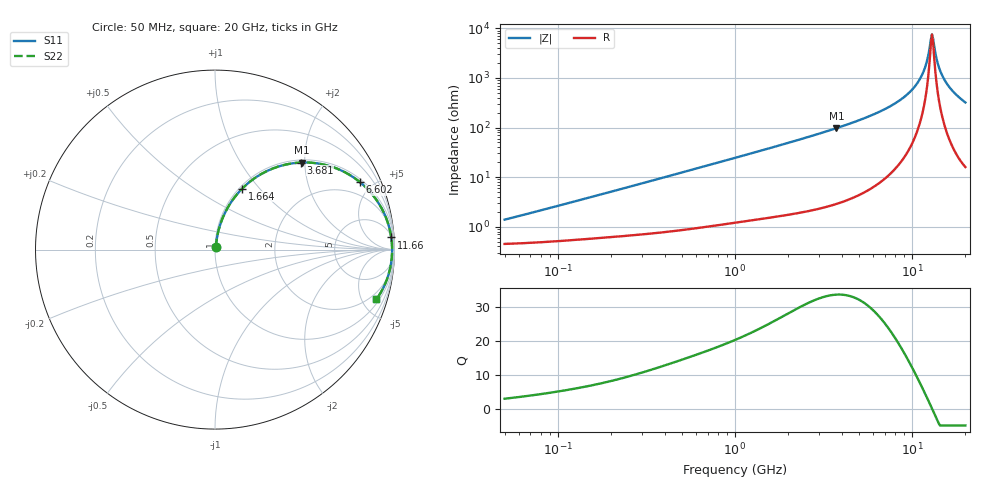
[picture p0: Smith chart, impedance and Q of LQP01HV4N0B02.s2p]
!Murata Part Number: LQP01HV4N0B02
!These Parameters are Measured in Series Mode Connection
!  o--[Z]--o
!Port1  Port2
!  o-------o
!Freq. Start=50[MHz] Stop=20[GHz], 401[Steps]
# Hz S RI R 50
!Freq.(Hz) S11(Real) S11(Imag) S21(Real) S21(Imag) S12(Real) S12(Imag) S22(Real) S22(Imag)
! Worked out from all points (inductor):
!   401 points, 50 MHz to 20 GHz, reference 50 ohm
!   read as one part in series: L = 4.16 nH near 52.3 MHz
!   highest Q = 33.8 at 3.736 GHz (marker M1), where L = 4.13 nH
!   self-resonance near 12.95 GHz
!   S11 on the Smith chart (normalised r, x): 50 MHz: 1.01, +0.03; 1.664 GHz: 1.03, +0.81; 3.681 GHz: 1.06, +1.91; 6.602 GHz: 1.16, +4.22; 11.66 GHz: 6, +28; 20 GHz: 1.32, -6.39
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5e7  0.00465 0.013  0.9954 -0.013  0.9954 -0.013  0.00465 0.013
1.364002e8  0.00671 0.0345  0.9933 -0.0345  0.9933 -0.0345  0.00671 0.0345
3.721004e8  0.0158 0.0903  0.9842 -0.0903  0.9842 -0.0903  0.0158 0.0903
1e9  0.0663 0.2253  0.9337 -0.2253  0.9337 -0.2253  0.0663 0.2253
1.664083e9  0.1515 0.3398  0.8485 -0.3398  0.8485 -0.3398  0.1515 0.3398
2.728004e9  0.3227 0.4521  0.6773 -0.4521  0.6773 -0.4521  0.3227 0.4521
3.680849e9  0.4772 0.4849  0.5228 -0.4849  0.5228 -0.4849  0.4772 0.4849
3.736399e9  0.4857 0.4852  0.5143 -0.4852  0.5143 -0.4852  0.4857 0.4852
4.966507e9  0.6524 0.461  0.3476 -0.461  0.3476 -0.461  0.6524 0.461
6.601595e9  0.8081 0.3757  0.1919 -0.3757  0.1919 -0.3757  0.8081 0.3757
7.442007e9  0.8631 0.323  0.1369 -0.323  0.1369 -0.323  0.8631 0.323
9.892087e9  0.9562 0.1689  0.0438 -0.1689  0.0438 -0.1689  0.9562 0.1689
1.082228e10  0.973 0.1143  0.027 -0.1143  0.027 -0.1143  0.973 0.1143
1.166392e10  0.982 0.0674  0.018 -0.0674  0.018 -0.0674  0.982 0.0674
1.201863e10  0.9844 0.0484  0.0156 -0.0484  0.0156 -0.0484  0.9844 0.0484
1.276073e10  0.9868 0.0101  0.0132 -0.0101  0.0132 -0.0101  0.9868 0.0101
1.295331e10  0.9869 0.000498  0.0131 -0.000498  0.0131 -0.000498  0.9869 0.000498
1.334722e10  0.9866 -0.0188  0.0134 0.0188  0.0134 0.0188  0.9866 -0.0188
1.417136e10  0.9836 -0.0575  0.0164 0.0575  0.0164 0.0575  0.9836 -0.0575
1.527346e10  0.9754 -0.1059  0.0246 0.1059  0.0246 0.1059  0.9754 -0.1059
1.721783e10  0.9515 -0.1827  0.0485 0.1827  0.0485 0.1827  0.9515 -0.1827
2e10  0.8997 -0.2764  0.1003 0.2764  0.1003 0.2764  0.8997 -0.2764
